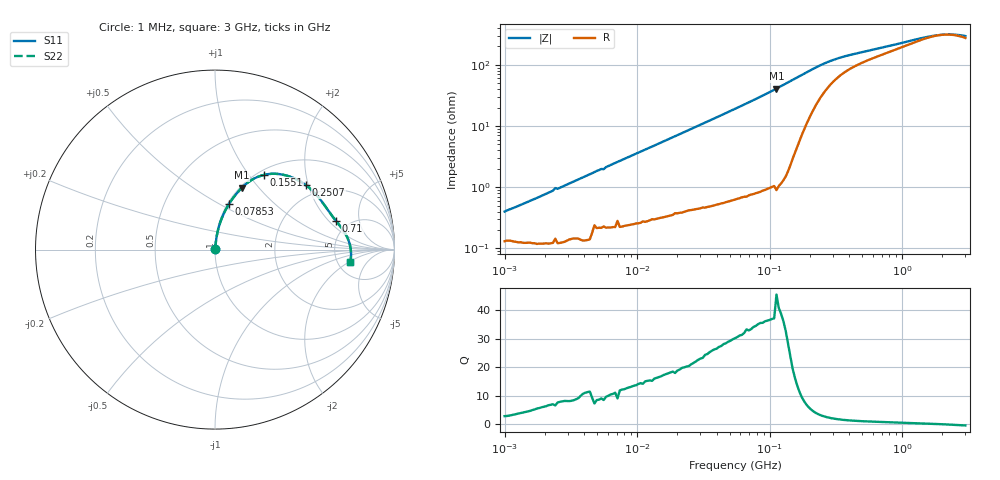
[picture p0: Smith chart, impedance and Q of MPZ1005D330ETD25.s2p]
! S-parameter Generated by TDK Corporation
! Copyright(C) 2018 TDK Corporation.
! All Rights Reserved.
! TDK P/N: MPZ1005D330ETD25 (Chip Bead)
! Property: |Z|=33¶ at 100MHz
! Size(LxWxT): 1x0.5x0.5mm, 0.039x0.02x0.02inches
! Model Type: s2p (Touchstone File Format Version 1.0)
! Frequency: DC=Yes Start=1MHz Stop=3000MHz 202points Log-sweep
! Model Generated on Aug. 6, 2018
! Port Assignments:
!  1 ---@@@--- 2
! Applicable Conditions:
!  Temperature = 25 degC
!  DC Bias Current = 0 A
!  Small Signal Operation
! Terms and conditions regarding TDK Simulation Models
! (1)This simulation model is being provided solely for informational purposes. Please refer to the specifications of the products in terms of detailed characteristics of such products.
! (2)In no event shall TDK Corporation of any of its subsidiaries be liable for any loss or damage arising, directly or indirectly,
!  From any information contained in this simulation model, including, but not limited to loss or damages arising from any inaccuracies, omissions or errors in connection with such information.
! (3)Any and all copyrights on this simulation model are owned by TDK Corporation.
!  Duplication or redistribution of this simulation model without prior written permission from TDK Corporation is prohibited.
! (4)This simulation model is subject to any modification or change without any prior notice.
! (5)Neither TDK Corporation nor any of its subsidiaries shall make any warranty, express or implied,
!  Including but not limited to the correctness, implied warranties of merchantability and fitness for a particular purpose with respect to this simulation models.
! (6)The use of this simulation model shall be deemed to have consented to the terms and conditions hereof.
# Hz S MA R 50
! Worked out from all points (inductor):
!   201 points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, 1 MHz to 3 GHz, reference 50 ohm
!   read as one part in series: L = 60.1 nH near 1.083 MHz
!   highest Q = 38.8 at 112.6 MHz (marker M1), where L = 57.7 nH
!   self-resonance near 2.075 GHz
!   S11 on the Smith chart (normalised r, x): 1 MHz: 1.00, +0.01; 78.53 MHz: 1.02, +0.55; 155.1 MHz: 1.07, +1.19; 250.7 MHz: 1.65, +1.93; 710 MHz: 3.94, +2.43; 3 GHz: 6.47, -2.16
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1000000  0.004002 70.6  0.9987 -0.2  0.9987 -0.2  0.004002 70.6
2055611  0.007786 80.6  0.9988 -0.4  0.9988 -0.4  0.007786 80.6
2317916  0.008788 81.4  0.9987 -0.5  0.9987 -0.5  0.008788 81.4
2412589  0.009682 80.9  0.9985 -0.5  0.9985 -0.5  0.009682 80.9
2511129  0.009383 82.0  0.9987 -0.5  0.9987 -0.5  0.009383 82.0
3900413  0.01445 83.8  0.9986 -0.8  0.9986 -0.8  0.01445 83.8
5372736  0.01981 82.6  0.9976 -1.1  0.9976 -1.1  0.01981 82.6
5592179  0.01966 82.2  0.9975 -1.1  0.9975 -1.1  0.01966 82.2
1.461624e7  0.05164 83.6  0.9956 -3.0  0.9956 -3.0  0.05164 83.6
3.00453e7  0.1038 81.6  0.9901 -6.0  0.9901 -6.0  0.1038 81.6
5.477226e7  0.1859 77.4  0.9764 -10.7  0.9764 -10.7  0.1859 77.4
7.852918e7  0.2638 73.1  0.957 -15.3  0.957 -15.3  0.2638 73.1
1.125904e8  0.3752 66.7  0.9188 -22.0  0.9188 -22.0  0.3752 66.7
1.550909e8  0.4988 56.6  0.8368 -29.9  0.8368 -29.9  0.4988 56.6
2.136344e8  0.5925 42.3  0.6891 -35.4  0.6891 -35.4  0.5925 42.3
2.507343e8  0.6211 35.3  0.6096 -36.0  0.6096 -36.0  0.6211 35.3
3.594878e8  0.6532 24.0  0.4832 -33.4  0.4832 -33.4  0.6532 24.0
7.099691e8  0.6926 13.4  0.3635 -26.2  0.3635 -26.2  0.6926 13.4
8.005644e8  0.701 12.0  0.3465 -24.9  0.3465 -24.9  0.701 12.0
1.855641e9  0.7532 1.6  0.2479 -4.7  0.2479 -4.7  0.7532 1.6
2.359433e9  0.7584 -1.8  0.2432 5.7  0.2432 5.7  0.7584 -1.8
3e9  0.7563 -5.4  0.2571 16.1  0.2571 16.1  0.7563 -5.4
